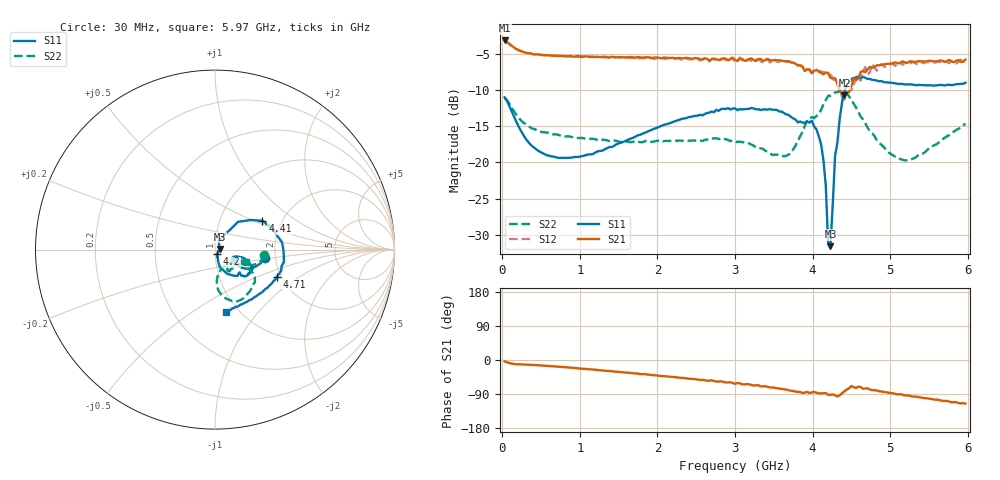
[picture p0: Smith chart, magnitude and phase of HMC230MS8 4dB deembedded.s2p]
!Hittite Microwave Corporation
!12 Elizabeth Drive
!Chelmsford, MA 01824
!Tel: 978-250-3343
!Fax: 978-250-3373
!Device: HMC230MS8, 0.75-2 GHz GaAs IC 3-bit Digital Attenuator in 8 lead plastic surface mount Mini Small Outline Package
!Misc: Room Temp Vdd = 5V , 4dB State.
# GHZ S DB R 50.0
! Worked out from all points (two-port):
!   199 points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, 30 MHz to 5.97 GHz, reference 50 ohm
!   highest |S21| = -3.20 dB at 30 MHz (marker M1); lowest = -10.7 dB at 4.41 GHz (marker M2)
!   |S21| within 3 dB of the highest: start of sweep to 3.718 GHz; 5.234 GHz to 5.818 GHz (584.5 MHz wide, 10.6 % of centre)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
!   lowest |S11| = -31.6 dB at 4.23 GHz (marker M3), VSWR 1.05, Z = 52.7 + j0.301 ohm
!   |S11| at or under -10 dB: start of sweep to 4.417 GHz
!   |S22| runs from -19.7 to -10.0 dB; largest |S21 - S12| = 0.054
!   S11 on the Smith chart (normalised r, x): 30 MHz: 1.76, -0.17; 4.2 GHz: 1.02, -0.05; 4.41 GHz: 1.60, +0.57; 4.71 GHz: 1.89, -0.67; 5.97 GHz: 0.88, -0.70
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0.03  -11.04 -9.2  -3.20 -3.5  -3.24 -3.4  -11.17 -6.3
0.15  -13.66 -31.0  -4.16 -10.5  -4.17 -10.2  -12.96 -22.4
0.45  -18.31 -33.2  -5.12 -13.6  -5.14 -13.7  -15.57 -28.3
1.02  -19.17 -22.3  -5.48 -22.8  -5.38 -22.8  -16.63 -39.0
2.04  -15.02 -17.4  -5.65 -42.0  -5.63 -41.8  -17.07 -49.0
3  -12.56 -30.4  -5.87 -62.6  -6.20 -62.1  -17.09 -57.2
3.66  -13.39 -42.7  -6.06 -78.1  -6.16 -77.0  -19.10 -38.2
3.99  -14.27 -49.7  -7.73 -85.6  -7.50 -85.3  -13.77 -31.2
4.08  -16.41 -63.0  -7.50 -87.9  -7.41 -87.4  -13.26 -30.5
4.14  -19.69 -74.5  -7.86 -87.8  -7.60 -89.1  -12.00 -31.9
4.17  -23.16 -75.2  -7.62 -87.3  -7.64 -89.4  -11.41 -34.5
4.2  -31.03 -65.3  -7.68 -91.8  -7.84 -91.4  -10.84 -39.1
4.23  -31.56 6.2  -8.35 -92.1  -7.94 -91.9  -10.80 -43.6
4.29  -19.10 55.9  -8.41 -93.1  -9.08 -94.7  -10.36 -50.1
4.41  -10.19 31.3  -10.74 -82.5  -11.37 -82.0  -10.07 -66.8
4.5  -8.51 6.2  -9.49 -68.8  -10.06 -72.9  -11.40 -79.7
4.65  -8.24 -17.5  -7.43 -75.7  -7.43 -68.7  -14.08 -86.8
4.71  -8.50 -23.8  -7.17 -74.8  -7.95 -79.4  -15.25 -86.8
4.77  -8.65 -28.6  -6.96 -79.4  -6.44 -77.4  -16.00 -85.5
4.98  -9.00 -40.8  -6.41 -86.5  -6.58 -84.4  -18.64 -74.3
5.31  -9.32 -55.1  -6.16 -96.7  -6.26 -96.4  -19.43 -46.8
5.97  -9.04 -79.8  -5.85 -115.2  -6.35 -111.2  -14.65 -22.6
